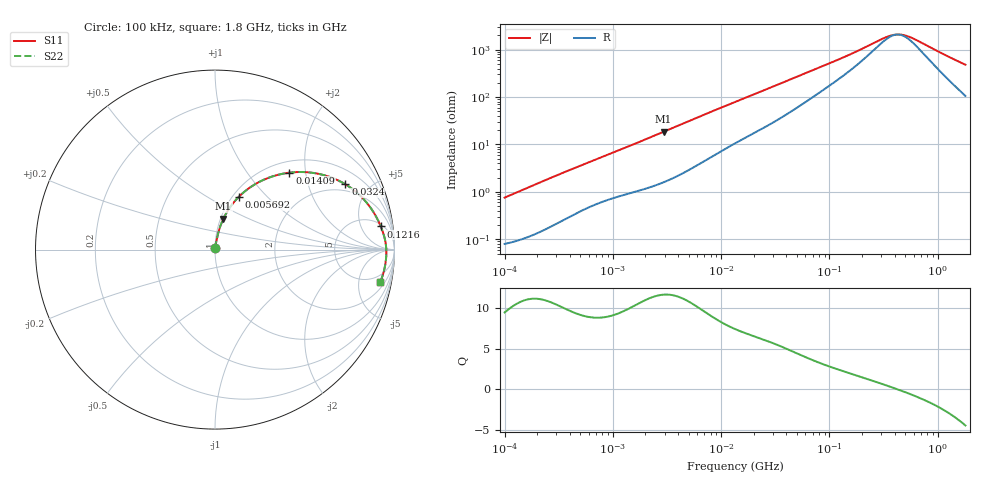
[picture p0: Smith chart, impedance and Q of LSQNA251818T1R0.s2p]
! LSQNA251818T1R0  S-PARAMETER MODEL  ( General Type )
! Model Generated by TAIYO YUDEN Corporation (http://www.ty-top.com)
! Version 2.0
! TAIYO YUDEN Control No. 100810NF25SB-FKC
! Copyright(c) 2007 TAIYO YUDEN CO.,LTD. All Rights Reserved.
! Product Description (link to TY-COMPAS)
! https://ds.yuden.co.jp/TYCOMPAS/or/detail?pn=LSQNA251818T1R0M&u=M
! Products Name : Inductors
! Characteristics :
!  Inductance : 1.0 uH , SRF(min) : 100 MHz , DC Resistance(max) : 0.078 Ohm
!  Rated Current : Saturation :1200 mA , Temp Rise : 1500 mA (40 degC)
!  Case Size : 2.5 x 1.8 / 0.098 x 0.071 [mm/inch] , Thickness : 1.8 / 0.071 [mm/inch]
!  (Conditions: Temperature = 25 degC , DC Bias Current/Voltage = 0A / 0V)
! External Node Assignments :
!  1  o---GGG---o  2
! GND o---------o GND
! Frequency Range : 0.1MHz  -  1800MHz  [ 402 STEP ]
# MHz S RI R 50
! Freq[MHz].  S11 Real  S11 Imag  S21 Real  S21 Imag  S12 Real  S12 Imag  S22 Real  S22 Imag
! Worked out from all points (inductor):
!   401 points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, 100 kHz to 1.8 GHz, reference 50 ohm
!   read as one part in series: L = 1.19 uH near 105 kHz
!   highest Q = 11.6 at 2.938 MHz (marker M1), where L = 1 uH
!   self-resonance near 422.6 MHz
!   S11 on the Smith chart (normalised r, x): 100 kHz: 1.00, +0.02; 5.692 MHz: 1.07, +0.70; 14.09 MHz: 1.22, +1.63; 32.4 MHz: 1.64, +3.51; 121.6 MHz: 6, +11; 1.8 GHz: 3.11, -9.38
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0.1  0.000852 0.0075  0.9991 -0.0075  0.9991 -0.0075  0.000852 0.0075
0.516129  0.00531 0.0361  0.9947 -0.0361  0.9947 -0.0361  0.00531 0.0361
1.277529  0.0153 0.0814  0.9847 -0.0814  0.9847 -0.0814  0.0153 0.0814
2.66389  0.0407 0.1589  0.9593 -0.1589  0.9593 -0.1589  0.0407 0.1589
2.938117  0.0472 0.1732  0.9528 -0.1732  0.9528 -0.1732  0.0472 0.1732
4.140031  0.0805 0.2315  0.9195 -0.2315  0.9195 -0.2315  0.0805 0.2315
5.692459  0.1321 0.2936  0.8679 -0.2936  0.8679 -0.2936  0.1321 0.2936
8.632747  0.2384 0.3727  0.7616 -0.3727  0.7616 -0.3727  0.2384 0.3727
13.41641  0.3955 0.426  0.6045 -0.426  0.6045 -0.426  0.3955 0.426
14.09005  0.4149 0.4287  0.5851 -0.4287  0.5851 -0.4287  0.4149 0.4287
20.85084  0.5717 0.4232  0.4283 -0.4232  0.4283 -0.4232  0.5717 0.4232
32.40491  0.7261 0.3641  0.2739 -0.3641  0.2739 -0.3641  0.7261 0.3641
46.79328  0.8174 0.2922  0.1826 -0.2922  0.1826 -0.2922  0.8174 0.2922
69.24595  0.8781 0.2165  0.1219 -0.2165  0.1219 -0.2165  0.8781 0.2165
121.6389  0.9237 0.1291  0.0763 -0.1291  0.0763 -0.1291  0.9237 0.1291
308.5485  0.9518 0.0286  0.0482 -0.0286  0.0482 -0.0286  0.9518 0.0286
357.3983  0.9533 0.0152  0.0467 -0.0152  0.0467 -0.0152  0.9533 0.0152
434.7684  0.9544 -0.00258  0.0456 0.00258  0.0456 0.00258  0.9544 -0.00258
479.5244  0.9547 -0.0115  0.0453 0.0115  0.0453 0.0115  0.9547 -0.0115
542.0029  0.9546 -0.023  0.0454 0.023  0.0454 0.023  0.9546 -0.023
1246.522  0.9414 -0.1184  0.0586 0.1184  0.0586 0.1184  0.9414 -0.1184
1800  0.9217 -0.1788  0.0783 0.1788  0.0783 0.1788  0.9217 -0.1788
